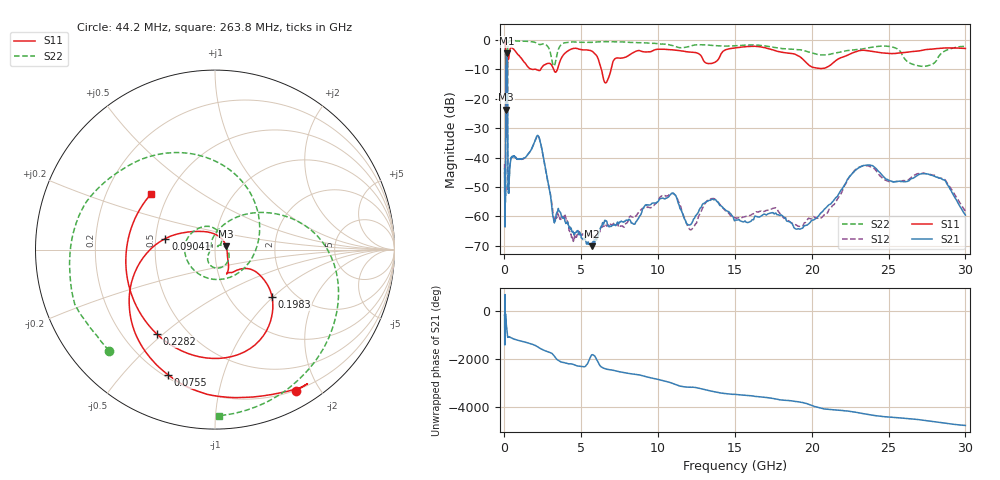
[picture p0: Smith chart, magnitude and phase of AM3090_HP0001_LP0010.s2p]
! Date/Time: Thu, Feb 28, 2019 1:53 PM
! Network Analyzer: Agilent Technologies E8364B Rev: A.07.50.67
! Sweep from 0.010 to 30.000 GHz, 1601 Points, Sweep Type: LOG
! Power Supply: 5.023 V, 0.002 A
# Hz S DB R 50
!freq MagS11 AngS11 MagS21 AngS21 MagS12 AngS12 MagS22 AngS22
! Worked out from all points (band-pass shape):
!   1601 points, 10 MHz to 30 GHz, reference 50 ohm
!   highest |S21| = -4.58 dB at 137 MHz (marker M1); lowest = -70.1 dB at 5.668 GHz (marker M2)
!   |S21| within 3 dB of the highest: 98.97 MHz to 183.9 MHz (84.9 MHz wide, 60 % of centre)
!   lowest |S11| = -23.8 dB at 98.44 MHz (marker M3), VSWR 1.14, Z = 56.6 + j2.04 ohm
!   |S11| at or under -10 dB: 2.038 GHz to 2.361 GHz (322.9 MHz wide, 14.7 % of centre); 3.201 GHz to 3.448 GHz (246.4 MHz wide, 7.41 % of centre); 6.308 GHz to 6.937 GHz (628.9 MHz wide, 9.5 % of centre)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
!   |S22| runs from -33.0 to -0.2 dB; largest |S21 - S12| = 0.014
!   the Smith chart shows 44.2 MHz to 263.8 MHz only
!   S11 on the Smith chart (normalised r, x): 44.2 MHz: 0.19, -1.71; 75.5 MHz: 0.21, -0.67; 90.41 MHz: 0.56, +0.08; 198.3 MHz: 1.55, -0.99; 228.2 MHz: 0.34, -0.48; 263.8 MHz: 0.40, +0.32
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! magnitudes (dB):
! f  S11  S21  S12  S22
! 10 MHz  -0.2  -43.9  -42.1  -0.6
! 38.04 MHz  -0.5  -61.7  -60.9  -1.4
! 44.2 MHz  -0.8  -60.1  -57.3  -1.8
! 75.5 MHz  -2.6  -45.1  -43.0  -4.9
! 90.41 MHz  -11.0  -14.7  -14.6  -15.5
! 98.44 MHz  -23.8  -7.8  -7.8  -15.7
! 137 MHz  -16.3  -4.6  -4.6  -25.8
! 144.7 MHz  -16.0  -4.6  -4.6  -21.3
! 177.7 MHz  -14.0  -6.4  -6.4  -31.6
! 198.3 MHz  -7.6  -16.2  -16.1  -10.6
! 228.2 MHz  -4.9  -49.6  -49.4  -1.6
! 263.8 MHz  -6.5  -51.9  -51.1  -0.7
! 550.5 MHz  -3.0  -39.7  -39.6  -0.2
! 2.084 GHz  -10.1  -33.0  -33.1  -1.0
! 3.269 GHz  -10.8  -61.8  -61.4  -8.5
! 5.668 GHz  -3.7  -70.1  -66.7  -0.8
! 6.619 GHz  -14.5  -61.7  -63.1  -0.6
! 7.926 GHz  -5.7  -61.3  -62.3  -0.8
! 10.7 GHz  -3.3  -53.3  -52.7  -1.6
! 19.41 GHz  -6.5  -64.0  -63.4  -3.5
! 23.48 GHz  -3.5  -42.6  -42.8  -2.9
! 30 GHz  -2.9  -59.6  -58.3  -2.2
